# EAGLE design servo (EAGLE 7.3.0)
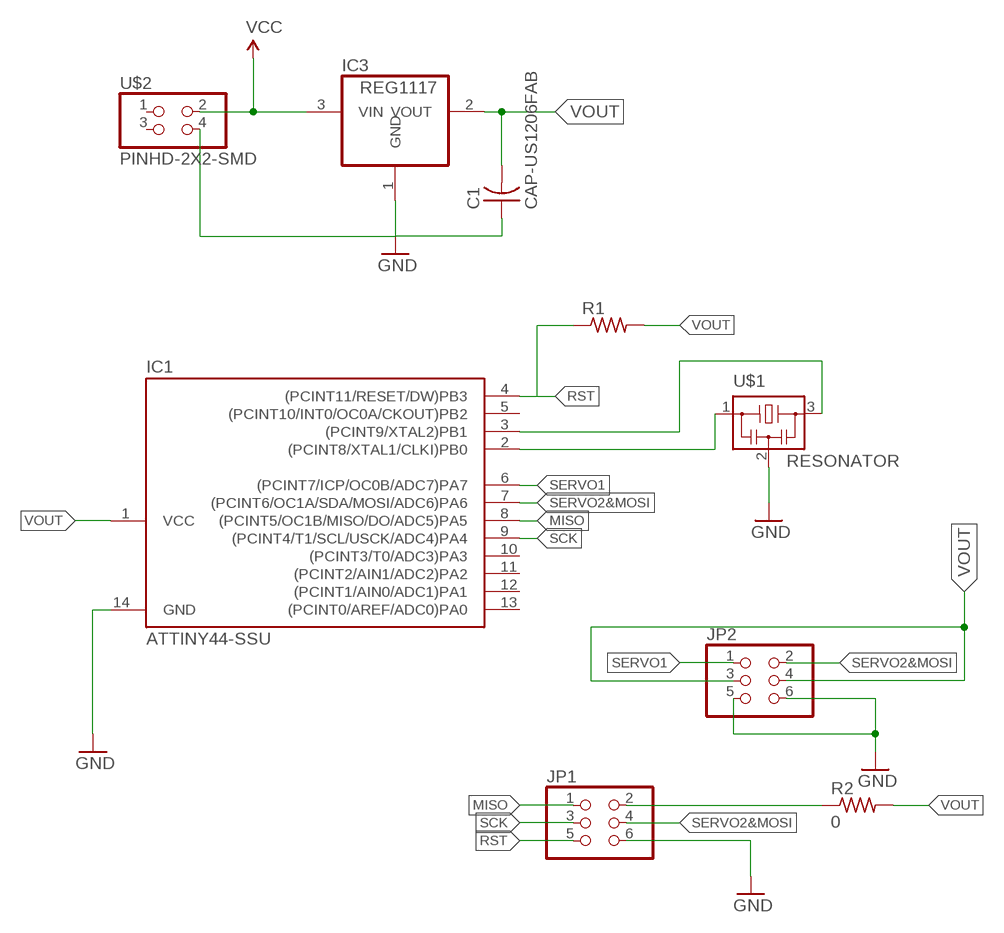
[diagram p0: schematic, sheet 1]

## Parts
C1  CAP-US1206FAB  [C1206FAB]
IC1  ATTINY44-SSU  [SOIC14]
IC3  REG1117  [SOT223]
JP1  PINHD-2X3-SMD  [2X03SMD]
JP2  PINHD-2X3-SMD  [2X03SMD]
R1  RES-US1206FAB  [R1206FAB]
R2  0  RES-US1206FAB  [R1206FAB]
U$1  RESONATOR  [EFOBM]
U$2  PINHD-2X2-SMD  [2X02SMD]

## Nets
GND: C1.1 IC1.14(GND) IC3.1(GND) JP1.6 JP2.5 JP2.6 U$1.2 U$2.4
MISO: IC1.8((PCINT5/OC1B/MISO/DO/ADC5)PA5) JP1.1
N$1: JP1.2 R2.1
N$11: IC1.2((PCINT8/XTAL1/CLKI)PB0) U$1.1
NO: IC1.3((PCINT9/XTAL2)PB1) U$1.3
RST: IC1.4((PCINT11/RESET/DW)PB3) JP1.5 R1.1
SCK: IC1.9((PCINT4/T1/SCL/USCK/ADC4)PA4) JP1.3
SERVO1: IC1.6((PCINT7/ICP/OC0B/ADC7)PA7) JP2.1
SERVO2&MOSI: IC1.7((PCINT6/OC1A/SDA/MOSI/ADC6)PA6) JP1.4 JP2.2
VCC: IC3.3(VIN) U$2.2
VOUT: C1.2 IC1.1(VCC) IC3.2(VOUT) JP2.3 JP2.4 R1.2 R2.2
Unconnected: IC1.5((PCINT10/INT0/OC0A/CKOUT)PB2) IC1.10((PCINT3/T0/ADC3)PA3) IC1.11((PCINT2/AIN1/ADC2)PA2) IC1.12((PCINT1/AIN0/ADC1)PA1) IC1.13((PCINT0/AREF/ADC0)PA0) U$2.1 U$2.3

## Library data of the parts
C1 = fab:CAP-US
IC1 = fab:ATTINY44
IC3 = burr-brown:REG1117: 800mA and 1A Low Dropout (LDO) Positive Regulator 1.8V, 2.5V, 2.85V, 3.3V, 5V, and Adj; MPN: REG1117; OC_FARNELL: 1097566; OC_NEWARK: 14P6981
JP1 JP2 = fab:PINHD-2X3-SMD: PIN HEADER
R1 R2 = fab:RES-US: Resistor (US Symbol)
U$1 = fab:RESONATOR
U$2 = fab:PINHD-2X2-SMD

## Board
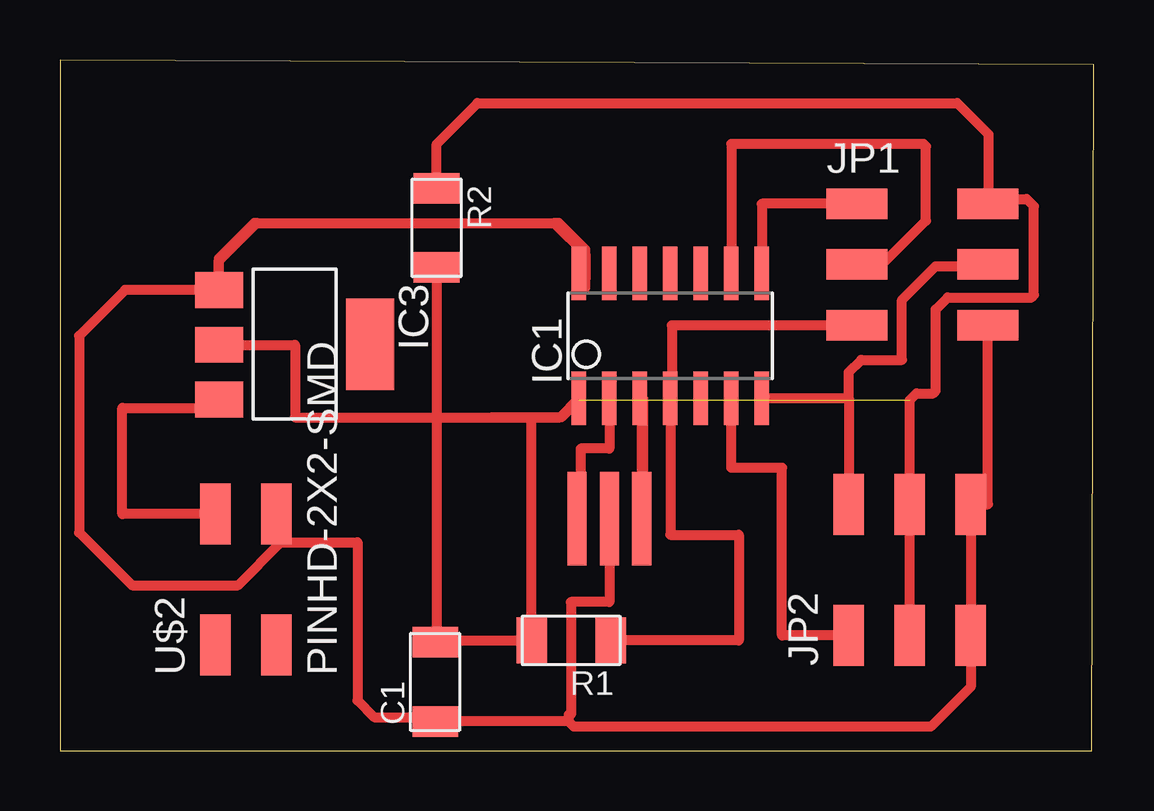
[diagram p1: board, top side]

Size 43.1 x 28.8 mm. Coordinates in mm from the lower left corner, seen from the top.
Outline: 0,0 43,0 43.1,28.6 0,28.8 0,0
Copper layers (1*16): Top 0.035mm / dielectric 1.5mm / Bottom 0.035mm
Design rules "default": minimum track width 10mil, minimum drill 24mil, track to track 8mil, track to pad 8mil, pad to pad 8mil, via to via 8mil, smd to smd 8mil, copper to edge 40mil, drill to drill 8mil, minimum pad ring 10mil, minimum via ring 8mil, stop-mask expansion 4mil, vias tented up to drill 0mil, thermal gap 10mil

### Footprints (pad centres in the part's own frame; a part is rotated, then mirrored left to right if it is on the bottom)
C1206FAB = smd 1.27 x 1.905: 1 -1.651,0; 2 1.651,0
SOIC14 = smd 0.61 x 2.21: 1 -3.81,-2.603; 2 -2.54,-2.603; 3 -1.27,-2.603; 4 0,-2.603; 5 1.27,-2.603; 6 2.54,-2.603; 7 3.81,-2.603; 8 3.81,2.603; 9 2.54,2.603; 10 1.27,2.603; 11 0,2.603; 12 -1.27,2.603; 13 -2.54,2.603; 14 -3.81,2.603
SOT223 = smd 1.499 x 2.007: 1 -2.261,-3.15; 2 0.025,-3.15; 3 2.311,-3.15 | smd 3.81 x 2.007: 4 0,3.15
2X03SMD = smd 2.54 x 1.27: 1 -2.54,2.54; 2 2.92,2.54; 3 -2.54,0; 4 2.92,0; 5 -2.54,-2.54; 6 2.92,-2.54
R1206FAB = smd 1.27 x 1.905: 1 -1.651,0; 2 1.651,0
EFOBM = smd 0.8 x 3.9: 1 -1.35,0; 2 0,0; 3 1.35,0
2X02SMD = smd 2.54 x 1.27: 1 -2.54,1.27; 2 2.92,1.27; 3 -2.54,-1.27; 4 2.92,-1.27

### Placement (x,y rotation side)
C1  15.64,2.87 90 top
IC1  25.44,17.3 0 top
IC3  9.78,16.95 270 top
JP1  35.76,20.27 0 top
JP2  35.42,7.35 90 top
R1  21.31,4.6 180 top
R2  15.7,21.8 270 top
U$1  22.9,9.68 0 top
U$2  7.75,6.95 90 top

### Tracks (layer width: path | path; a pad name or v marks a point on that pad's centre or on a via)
GND
  Top 0.406: JP2.6 JP2.5 | 23,9.68 U$1.2 22.9,6.2 21.3,6.2 21.3,1.5 21.2,1.5 21.2,1.22 | JP2.6 38.68,10.27 JP1.6 | U$2.4 9.21,8.69 | 8.2,22 8.1,22 6.63,20.53 IC3.1 2.71,19.21 0.8,17.3 0.8,9.1 3,6.9 7.42,6.9 9.21,8.69 | 8.2,22 20.6,22 | 20.6,22 21.9,20.7 | 21.9,20.7 21.9,19.63 | 21.9,19.3 21.9,19.63 | 21.9,19.63 IC1.14 | 21.2,1.22 C1.1 | C1.1 15.64,1.17 | 21.9,20.7 21.9,20.9 20.8,22 20.6,22 | 8.2,22 6.6,20.4 6.6,19.3 6.5,19.2 | 9.21,8.69 12.38,8.69 12.4,8.7 12.4,2.1 13.1,1.4 15.46,1.4 C1.1 | JP2.6 37.96,2.66 36.3,1 21.42,1 21.2,1.22
MISO
  Top 0.406: JP1.1 29.25,22.81 IC1.8
N$1
  Top 0.406: R2.1 15.7,25.3 17.4,27 37.4,27 38.7,25.7 38.7,22.83 JP1.2
N$11
  Top 0.406: IC1.2 22.9,12.6 21.7,12.6 21.7,10.5 21.4,10.5 21.4,9.68 U$1.1
NO
  Top 0.406: 24.3,10.9 24.3,14.7 IC1.3 24.25,14.7 U$1.3
RST
  Top 0.406: JP1.5 25.5,17.73 25.5,15.2 25.44,15.2 IC1.4 25.44,9 28.3,9 28.3,4.6 R1.1
SCK
  Top 0.406: IC1.9 27.98,25.3 36,25.3 36.1,25.2 36.1,22.1 34.27,20.27 JP1.3
SERVO1
  Top 0.406: JP2.1 30.1,4.81 30.1,11.8 27.98,11.8 IC1.6
SERVO2&MOSI
  Top 0.406: IC1.7 32.88,14.7 | 32.88,14.7 JP2.2 | JP1.4 38.61,20.2 36.5,20.2 35.1,18.8 35.1,16.3 33.4,16.3 32.88,15.78 32.88,14.7
VCC
  Top 0.406: U$2.2 2.6,9.87 2.6,14.3 6.16,14.3 IC3.3
VOUT  (1 unrouted)
  Top 0.406: 35.5,4.81 JP2.3 JP2.4 35.42,14.62 35.7,14.9 36.4,14.9 36.5,15 36.5,18.4 37,18.9 40.5,18.9 40.6,19 40.6,22.7 40.3,23 38.87,23 | IC3.2 9.8,16.93 9.8,13.9 19.66,13.9 | 19.66,13.9 20.83,13.9 IC1.1 21.63,14.63 20.9,13.9 18,13.9 | 19.66,13.9 R1.2 15.64,4.6 C1.2 15.7,4.58 R2.2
